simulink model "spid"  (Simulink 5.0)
settings: Solver=ode4  SolverMode=SingleTasking  StartTime=0.0  StopTime=100  FixedStep=2  RelTol=1e-3  AbsTol=1e-6

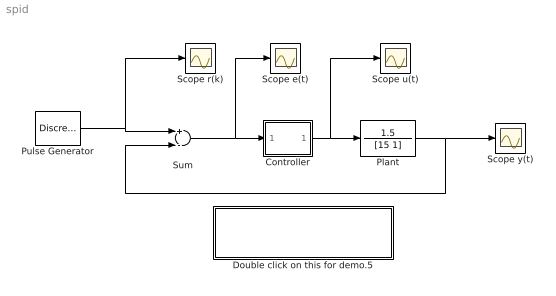
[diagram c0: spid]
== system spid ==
  Controller : Subsystem  mask(Controller){P=0.1, I=1.5, D=2}
      mask prompts: P "Proportional :"; I "Integral :"; D "Derivative :"
      mask help: Enter expressions for proportional, integral, and derivative terms.
      mask init:
      | P=@1; I=@2; D=@3;
  Double click on this for demo.5 : Subsystem
  Plant : TransferFcn  Numerator=1.5  Denominator=[15 1]
  Pulse Generator : DiscretePulseGenerator  Period=250  PulseWidth=50  SampleTime=2
  Scope e(t) : Scope
  Scope r(k) : Scope
  Scope u(t) : Scope
  Scope y(t) : Scope
  Sum : Sum  Inputs=+-
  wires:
  Controller/1(Out_1) -> Plant/1, Scope u(t)/1
  Pulse Generator/1 -> Sum/1, Scope r(k)/1
  Plant/1 -> Scope y(t)/1, Sum/2
  Sum/1 -> Controller/1(In_1), Scope e(t)/1

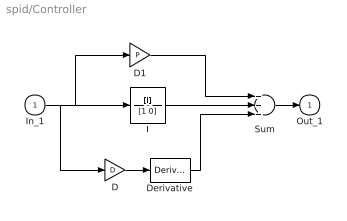
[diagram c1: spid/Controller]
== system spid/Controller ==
  In_1 : Inport
  D : Gain  Gain=D
  D1 : Gain  Gain=P
  Derivative : Derivative
  I : TransferFcn  Numerator=[I]  Denominator=[1 0]
  Sum : Sum  Inputs=+++
  Out_1 : Outport  InitialOutput=0
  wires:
  In_1/1 -> D1/1, I/1, D/1
  Sum/1 -> Out_1/1
  D/1 -> Derivative/1
  Derivative/1 -> Sum/3
  I/1 -> Sum/2
  D1/1 -> Sum/1

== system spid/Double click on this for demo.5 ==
